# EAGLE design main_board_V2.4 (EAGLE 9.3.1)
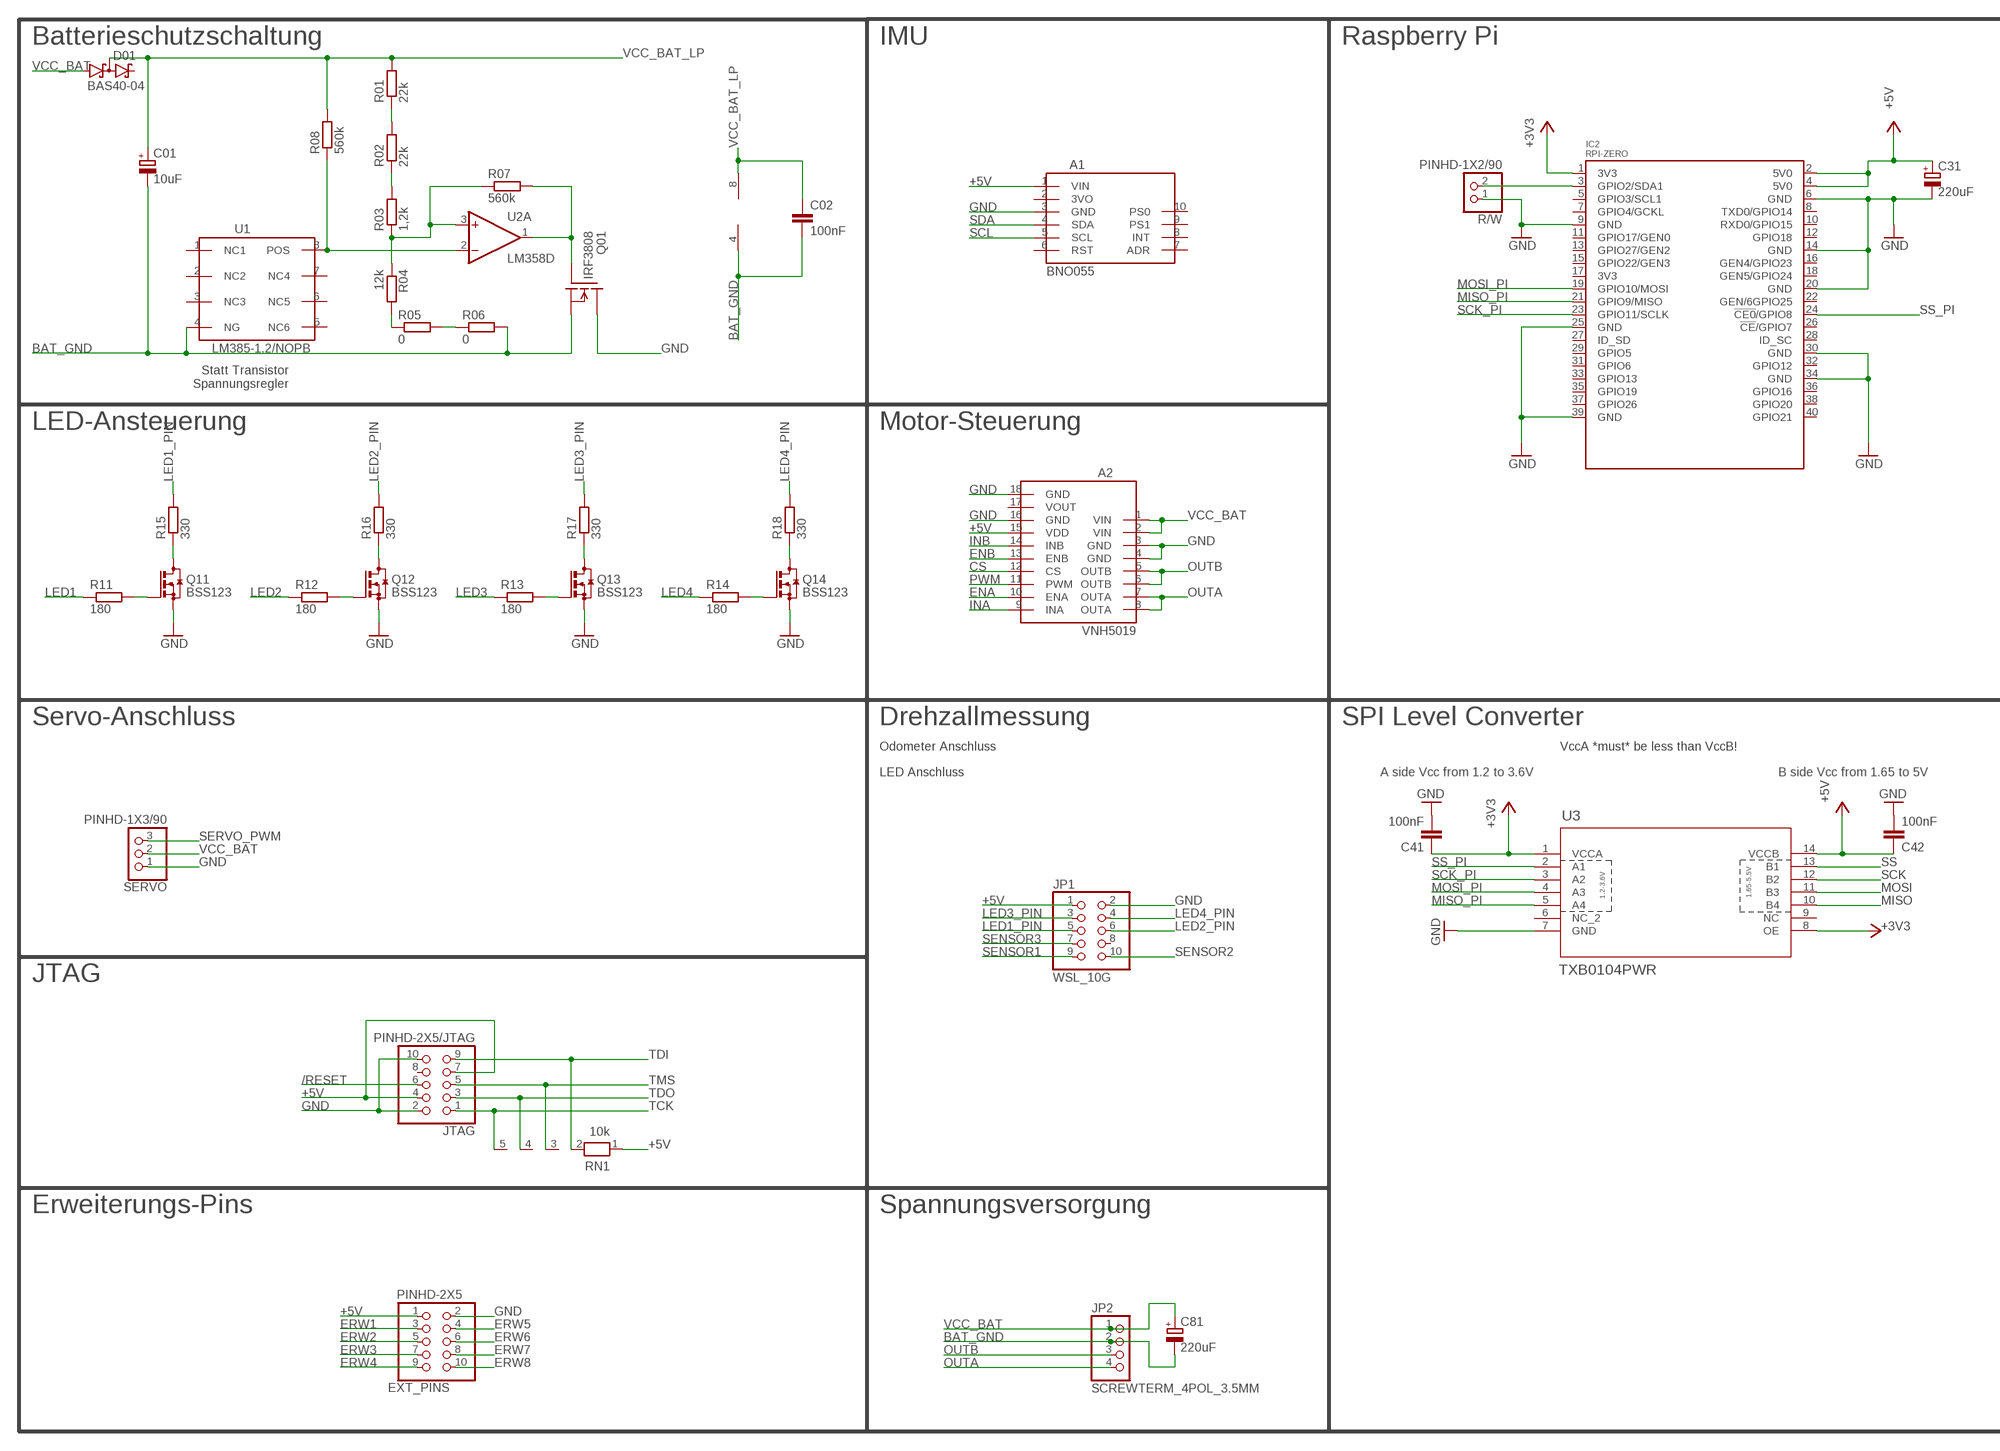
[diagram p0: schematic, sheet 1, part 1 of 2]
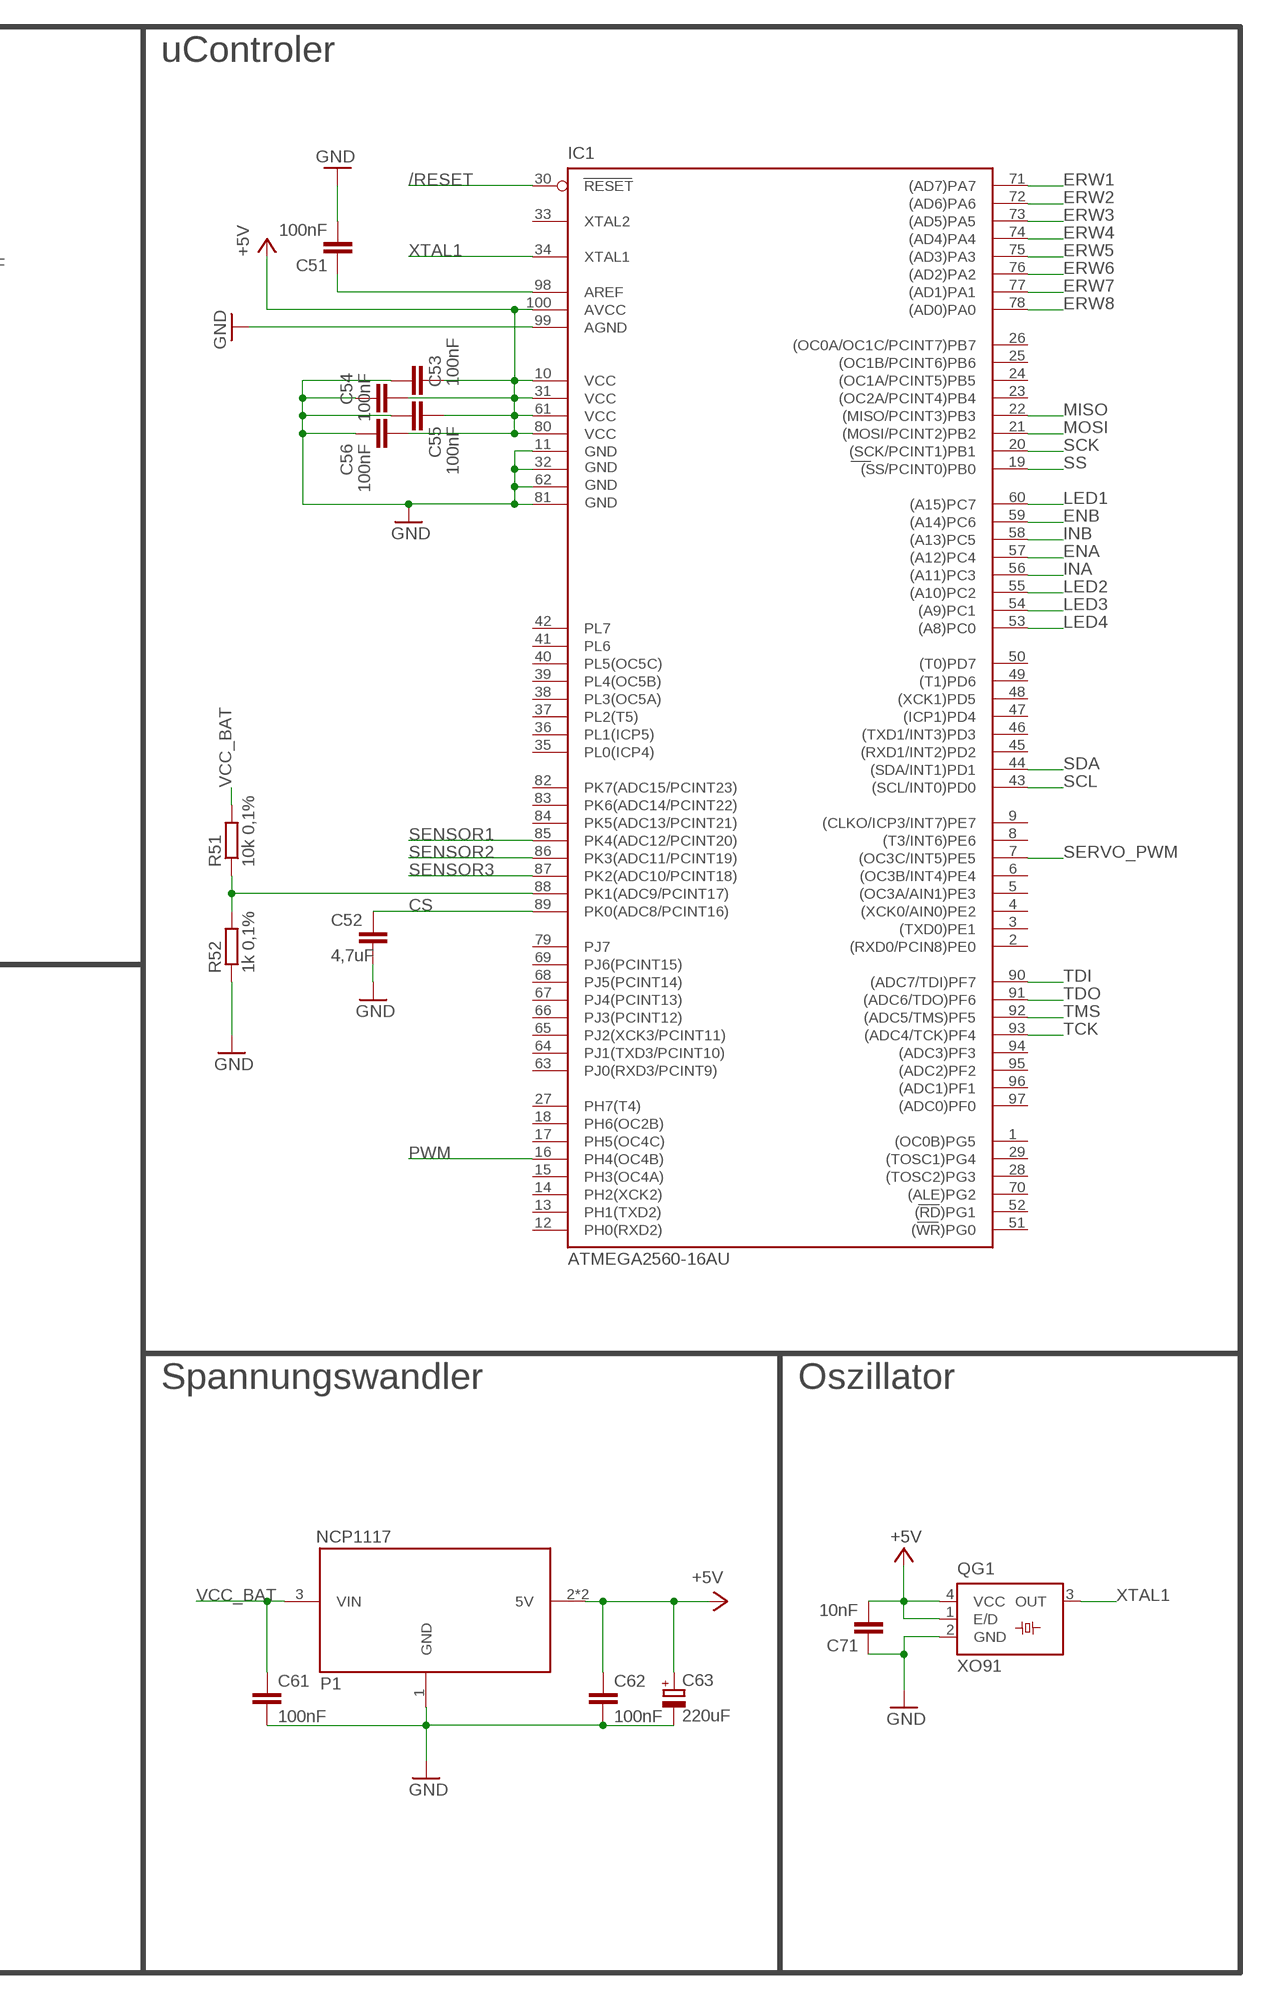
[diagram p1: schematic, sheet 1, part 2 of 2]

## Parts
A1  BNO055  [BNO055]
A2  VNH5019  [VNH5019]
C01  10uF  CPOL/4X5,8  [UD-4X5,8_NICHICON]
C02  100nF  C-EUC0805  [C0805]
C31  220uF  CPOL/6,3X7,7  [UD-6,3X5,8_NICHICON]
C41  100nF  C-EUC0805  [C0805]
C42  100nF  C-EUC0805  [C0805]
C51  100nF  C-EUC0805  [C0805]
C52  4,7uF  C-EUC0805  [C0805]
C53  100nF  C-EUC0805  [C0805]
C54  100nF  C-EUC0805  [C0805]
C55  100nF  C-EUC0805  [C0805]
C56  100nF  C-EUC0805  [C0805]
C61  100nF  C-EUC0805  [C0805]
C62  100nF  C-EUC0805  [C0805]
C63  220uF  CPOL/6,3X7,7  [UD-6,3X5,8_NICHICON]
C71  10nF  C-EUC0805  [C0805]
C81  220uF  CPOL/6,3X7,7  [UD-6,3X5,8_NICHICON]
D01  BAS40-04  [SOT23]
EXT_PINS  PINHD-2X5  [2X05]
IC1  ATMEGA2560-16AU  [TQFP100]
IC2  RPI-ZERO  [RASPBERRYPI_ZERO]
JP1  WSL_10G  [WSL_10G]
JP2  SCREWTERM_4POL_3.5MM  [SCREWTERM_4POS_3.5MM]
JTAG  PINHD-2X5/JTAG  [2X05/JTAG]
P1  NCP1117  [SOT223]
Q01  IRF3808  [TO220]
Q11  BSS123  [SOT23]
Q12  BSS123  [SOT23]
Q13  BSS123  [SOT23]
Q14  BSS123  [SOT23]
QG1  XO91  [SM77H]
R01  22k  R-EUR0805  [R0805]
R02  22k  R-EUR0805  [R0805]
R03  1,2k  R-EUR0805  [R0805]
R04  12k  R-EUR0805  [R0805]
R05  0  R-EUR0805  [R0805]
R06  0  R-EUR0805  [R0805]
R07  560k  R-EUR0805  [R0805]
R08  560k  R-EUR0805  [R0805]
R11  180  R-EUR0805  [R0805]
R12  180  R-EUR0805  [R0805]
R13  180  R-EUR0805  [R0805]
R14  180  R-EUR0805  [R0805]
R15  330  R-EUR0805  [R0805]
R16  330  R-EUR0805  [R0805]
R17  330  R-EUR0805  [R0805]
R18  330  R-EUR0805  [R0805]
R51  10k 0,1%  R-EUR0805  [R0805]
R52  1k 0,1%  R-EUR0805  [R0805]
R/W  PINHD-1X2/90  [1X02/90]
RN1  10k  RN04  [RN04]
SERVO  PINHD-1X3/90  [1X03/90]
U1  LM385-1.2/NOPB  [SO08]
U2  LM358D  [SO08]
U3  TXB0104PWR  [PW14]

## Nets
+3V3: C41.1 IC2.1(3V3) U3.1(VCCA) U3.8(OE)
+5V: A1.1(VIN) A2.15(VDD) C31.+ C42.1 C53.1 C54.1 C55.1 C56.1 C62.1 C63.+ C71.2 EXT_PINS.1 IC1.10(VCC) IC1.31(VCC1) IC1.61(VCC2) IC1.80(VCC3) IC1.100(AVCC) IC2.2(5V0) IC2.4(5V0) JP1.1 JTAG.4 JTAG.7 P1.2(5V) P1.4(5V) QG1.1(E/D) QG1.4(VCC) RN1.1 U3.14(VCCB)
/RESET: IC1.30(RESET) JTAG.6
BAT_GND: C01.- C02.2 C81.- JP2.2 Q01.3(S) R06.2 U1.4(NG) U2.4(P:V-)
CS: A2.12(CS) C52.1 IC1.89(PK0(ADC8/PCINT16))
ENA: A2.10(ENA) IC1.57((A12)PC4)
ENB: A2.13(ENB) IC1.59((A14)PC6)
ERW1: EXT_PINS.3 IC1.71((AD7)PA7)
ERW2: EXT_PINS.5 IC1.72((AD6)PA6)
ERW3: EXT_PINS.7 IC1.73((AD5)PA5)
ERW4: EXT_PINS.9 IC1.74((AD4)PA4)
ERW5: EXT_PINS.4 IC1.75((AD3)PA3)
ERW6: EXT_PINS.6 IC1.76((AD2)PA2)
ERW7: EXT_PINS.8 IC1.77((AD1)PA1)
ERW8: EXT_PINS.10 IC1.78((AD0)PA0)
GND: A1.3(GND) A2.3(GND) A2.4(GND) A2.16(GND) A2.18(GND) C31.- C41.2 C42.2 C51.2 C52.2 C53.2 C54.2 C55.2 C56.2 C61.2 C62.2 C63.- C71.1 EXT_PINS.2 IC1.11(GND) IC1.32(GND1) IC1.62(GND2) IC1.81(GND3) IC1.99(AGND) IC2.6(GND) IC2.9(GND) IC2.14(GND) IC2.20(GND) IC2.25(GND) IC2.30(GND) IC2.34(GND) IC2.39(GND) JP1.2 JTAG.2 JTAG.10 P1.1(GND) Q01.2(D) Q11.2(S) Q12.2(S) Q13.2(S) Q14.2(S) QG1.2(GND) R52.1 R/W.1 SERVO.1 U3.7(GND)
INA: A2.9(INA) IC1.56((A11)PC3)
INB: A2.14(INB) IC1.58((A13)PC5)
LED1: IC1.60((A15)PC7) R11.1
LED1_PIN: JP1.5 R15.2
LED2: IC1.55((A10)PC2) R12.1
LED2_PIN: JP1.6 R16.2
LED3: IC1.54((A9)PC1) R13.1
LED3_PIN: JP1.3 R17.2
LED4: IC1.53((A8)PC0) R14.1
LED4_PIN: JP1.4 R18.2
MISO: IC1.22((MISO/PCINT3)PB3) U3.10(B4)
MISO_PI: IC2.21(GPIO9/MISO) U3.5(A4)
MOSI: IC1.21((MOSI/PCINT2)PB2) U3.11(B3)
MOSI_PI: IC2.19(GPIO10/MOSI) U3.4(A3)
N$1: R05.2 R06.1
N$2: R03.1 R04.1 R07.1 U2.3(A:+IN)
N$3: R08.1 U1.8(POS) U2.2(A:-IN)
N$5: R01.1 R02.2
N$6: Q01.1(G) R07.2 U2.1(A:OUT)
N$7: R02.1 R03.2
N$8: IC2.3(GPIO2/SDA1) R/W.2
N$9: Q11.1(G) R11.2
N$10: Q12.1(G) R12.2
N$11: C51.1 IC1.98(AREF)
N$12: R04.2 R05.1
N$13: Q13.1(G) R13.2
N$14: Q14.1(G) R14.2
N$18: Q11.3(D) R15.1
N$19: Q12.3(D) R16.1
N$26: Q13.3(D) R17.1
N$29: Q14.3(D) R18.1
N$30: IC1.88(PK1(ADC9/PCINT17)) R51.1 R52.2
OUTA: A2.7(OUTA) A2.8(OUTA) JP2.4
OUTB: A2.5(OUTB) A2.6(OUTB) JP2.3
PWM: A2.11(PWM) IC1.16(PH4(OC4B))
SCK: IC1.20((SCK/PCINT1)PB1) U3.12(B2)
SCK_PI: IC2.23(GPIO11/SCLK) U3.3(A2)
SCL: A1.5(SCL) IC1.43((SCL/INT0)PD0)
SDA: A1.4(SDA) IC1.44((SDA/INT1)PD1)
SENSOR1: IC1.85(PK4(ADC12/PCINT20)) JP1.9
SENSOR2: IC1.86(PK3(ADC11/PCINT19)) JP1.10
SENSOR3: IC1.87(PK2(ADC10/PCINT18)) JP1.7
SERVO_PWM: IC1.7((OC3C/INT5)PE5) SERVO.3
SS: IC1.19((SS/PCINT0)PB0) U3.13(B1)
SS_PI: IC2.24(!CE0!/GPIO8) U3.2(A1)
TCK: IC1.93((ADC4/TCK)PF4) JTAG.1 RN1.5
TDI: IC1.90((ADC7/TDI)PF7) JTAG.9 RN1.2
TDO: IC1.91((ADC6/TDO)PF6) JTAG.3 RN1.4
TMS: IC1.92((ADC5/TMS)PF5) JTAG.5 RN1.3
VCC_BAT: A2.1(VIN) A2.2(VIN) C61.1 C81.+ D01.1(A1) JP2.1 P1.3(VIN) R51.2 SERVO.2
VCC_BAT_LP: C01.+ C02.1 D01.3(C1A2) R01.2 R08.2 U2.8(P:V+)
XTAL1: IC1.34(XTAL1) QG1.3(OUT)
Unconnected: A1.2(3VO) A1.6(RST) A1.7(ADR) A1.8(INT) A1.9(PS1) A1.10(PS0) A2.17(VOUT) D01.2(C2) IC1.1((OC0B)PG5) IC1.2((RXD0/PCIN8)PE0) IC1.3((TXD0)PE1) IC1.4((XCK0/AIN0)PE2) IC1.5((OC3A/AIN1)PE3) IC1.6((OC3B/INT4)PE4) IC1.8((T3/INT6)PE6) IC1.9((CLKO/ICP3/INT7)PE7) IC1.12(PH0(RXD2)) IC1.13(PH1(TXD2)) IC1.14(PH2(XCK2)) IC1.15(PH3(OC4A)) IC1.17(PH5(OC4C)) IC1.18(PH6(OC2B)) IC1.23((OC2A/PCINT4)PB4) IC1.24((OC1A/PCINT5)PB5) IC1.25((OC1B/PCINT6)PB6) IC1.26((OC0A/OC1C/PCINT7)PB7) IC1.27(PH7(T4)) IC1.28((TOSC2)PG3) IC1.29((TOSC1)PG4) IC1.33(XTAL2) IC1.35(PL0(ICP4)) IC1.36(PL1(ICP5)) IC1.37(PL2(T5)) IC1.38(PL3(OC5A)) IC1.39(PL4(OC5B)) IC1.40(PL5(OC5C)) IC1.41(PL6) IC1.42(PL7) IC1.45((RXD1/INT2)PD2) IC1.46((TXD1/INT3)PD3) IC1.47((ICP1)PD4) IC1.48((XCK1)PD5) IC1.49((T1)PD6) IC1.50((T0)PD7) IC1.51((WR)PG0) IC1.52((RD)PG1) IC1.63(PJ0(RXD3/PCINT9)) IC1.64(PJ1(TXD3/PCINT10)) IC1.65(PJ2(XCK3/PCINT11)) IC1.66(PJ3(PCINT12)) IC1.67(PJ4(PCINT13)) IC1.68(PJ5(PCINT14)) IC1.69(PJ6(PCINT15)) IC1.70((ALE)PG2) IC1.79(PJ7) IC1.82(PK7(ADC15/PCINT23)) IC1.83(PK6(ADC14/PCINT22)) IC1.84(PK5(ADC13/PCINT21)) IC1.94((ADC3)PF3) IC1.95((ADC2)PF2) IC1.96((ADC1)PF1) IC1.97((ADC0)PF0) IC2.5(GPIO3/SCL1) IC2.7(GPIO4/GCKL) IC2.8(TXD0/GPIO14) IC2.10(RXD0/GPIO15) IC2.11(GPIO17/GEN0) IC2.12(GPIO18) IC2.13(GPIO27/GEN2) IC2.15(GPIO22/GEN3) IC2.16(GEN4/GPIO23) IC2.17(3V3) IC2.18(GEN5/GPIO24) IC2.22(GEN/6GPIO25) IC2.26(!CE!/GPIO7) IC2.27(ID_SD) IC2.28(ID_SC) IC2.29(GPIO5) IC2.31(GPIO6) IC2.32(GPIO12) IC2.33(GPIO13) IC2.35(GPIO19) IC2.36(GPIO16) IC2.37(GPIO26) IC2.38(GPIO20) IC2.40(GPIO21) JP1.8 JTAG.8 U1.1(NC1) U1.2(NC2) U1.3(NC3) U1.5(NC6) U1.6(NC5) U1.7(NC4) U2.5(B:+IN) U2.6(B:-IN) U2.7(B:OUT) U3.6(NC_2) U3.9(NC)

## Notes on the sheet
- Batterieschutzschaltung | IMU | Raspberry Pi | uControler
- Statt Transistor
  Spannungsregler
- LED-Ansteuerung | Motor-Steuerung
- Servo-Anschluss | Drehzallmessung | SPI Level Converter
- Odometer Anschluss | VccA *must* be less than VccB!
- LED Anschluss | A side Vcc from 1.2 to 3.6V | B side Vcc from 1.65 to 5V
- JTAG
- Spannungswandler | Oszillator
- Erweiterungs-Pins | Spannungsversorgung

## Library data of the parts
A1 = embedded:BNO055: BREAKOUT BOARD Adafruit BNO055 Absolute Orientation Sensor https://learn.adafruit.com/adafruit-bno055-absolute-orientation-sensor/overview; DATASHEET: https://cdn-learn.adafruit.com/downloads/pdf/adafruit-bno055-absolute-orientation-sensor.pdf; DESCR: Acceleration Sensor Development Tools Adafruit 9-DOF Absolute Orientation IMU Fusion Breakout - BNO055; MF: Adafruit; MF_PN: 2472; MOUSER_NO: 485-2472; PURCHASE: https://www.reichelt.de/development-boards-sensor-with-different-functions-debo-sens-combi-p235479.html?PROVID=2788&gclid=EAIaIQobChMIppaP2Nqd4gIVA853Ch3mIQILEAYYASABEgKn7_D_BwE&&r=1; REICHELT_NO: DEBO SENS COMBI; UNIT_PRICE: 30.52
A2 = embedded:VNH5019: Pololu VNH5019 Motor Driver Carrier Operating voltage: 5.5 – 24 V1 Output current: 12 A continuous (30 maximum) 3V-compatible inputs PWM operation up to 20 kHz, which is ultrasonic and allows for quieter motor operation Current sense output proportional to motor current (approx. 140 mV/A; only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; DATASHEET: https://www.st.com/content/ccc/resource/technical/document/data_brief/3b/bf/c3/13/d5/b2/4c/b0/DM00101248.pdf/files/DM00101248.pdf/jcr:content/translations/en.DM00101248.pdf; DESCR: VNH5019 Motor Controller/Driver Power Management Evaluation Board; DIGIKEY_NO: 497-14839-ND; MF: Pololu; MF_PN: 1451; PURCHASE: https://www.digikey.de/product-detail/de/stmicro/EVAL-VNH5019-P1/497-14839-ND/4869482?utm_adgroup=Dev+Boards+and+Kits&mkwid=siS2m191I&pcrid=218211101233&pkw=&pmt=&pdv=c&productid=4869482&slid=&gclid=CjwKCAjw2cTmBRAVEiwA8YMgzaipRkISnCfVdTSSKNDcojFwUwpzQeKwWGZWYQUEEXtJxoFNqy7q1BoC5-sQAvD_BwE; UNIT_PRICE: 33.42
C01 = embedded:CPOL: Aluminum Electrolytic Capacitors; DATASHEET: https://industrial.panasonic.com/cdbs/www-data/pdf/RDE0000/ABA0000C1175.pdf; DESCR: Aluminium Electrolytic Capacitors - SMD FK 35VDC 10uF SMD 4x5.8; FARNELL_NO: 1244420; MF: Panasonic; MF_PN: EEEFKV100UAR; PACKAGE: 4x5.8; PURCHASE: https://de.farnell.com/panasonic/eeefkv100uar/kondensator-10-f-35v-radial-smd/dp/1244420; SIZE: 4x5.8mm; UNIT_PRICE: 0.376
C02 C41 C42 C51-C56 C61 C62 C71 = embedded:C-EU: Capacitor; DESCR: SMD Capacitor; PACKAGE: C0805; SIZE: 0805in
C31 C63 C81 = embedded:CPOL: Aluminum Electrolytic Capacitors; DATASHEET: https://industrial.panasonic.com/cdbs/www-data/pdf/RDE0000/ABA0000C1175.pdf; DESCR: Aluminium Electrolytic Capacitors - SMD FK 16VDC 10uF SMD 6.3x7.7; FARNELL_NO: 2254321; MF: Panasonic; MF_PN: EEEFKC221XAP; PACKAGE: 6.3x7.7; PURCHASE: https://de.farnell.com/panasonic/eeefkc221xap/kondensator-220-f-16v-radial-smd/dp/2254321; SIZE: 6.3x7.7mm; UNIT_PRICE: 0.48
D01 = embedded:BAS40-04: Silicon Schottky Diodes General-purpose diode for high-speed switching; DATASHEET: https://www.onsemi.com/pub/Collateral/BAS40-04LT1-D.PDF; DESCR: Schottky Diodes & Rectifiers 40V 225mW Dual; FARNELL_NO: 2317418; MF: ON Semiconductor; MF_PN: BAS40-04LT1G; MOUSER_NO: 863-BAS40-04LT1G; PACKAGE: SOT-23-3; PURCHASE: https://de.farnell.com/on-semiconductor/bas40-04lt1g/schottky-diode-40ma-40v-sot-23/dp/2317418; UNIT_PRICE: 0.236
EXT_PINS = embedded:PINHD-2X5: PIN HEADER; ANGLE: Straight; DESCR: Pin Header 2X5 0DEG; PACKAGE: Pin Header; PITCH: 2.54mm; POS: 10; ROWS: 2
IC1 = embedded:ATMEGA*: MICROCONTROLLER 64/128/256 Kbytes FLASH 4 Kbytes EEPROM 8 Kbytes SRAM 86 General Purpose I/O pins 12-channels16-bit PWM 4 x Serial USARTs 16-channels 10-bit A/D; DATASHEET: http://ww1.microchip.com/downloads/en/DeviceDoc/Atmel-2549-8-bit-AVR-Microcontroller-ATmega640-1280-1281-2560-2561_datasheet.pdf; DESCR: 8-bit Microcontrollers - MCU 256kB Flash 4kB EEPROM 86 I/O Pins; FARNELL_NO: 1288330; MF: Atmel; MF_PN: ATMEGA2560-16AU; MOUSER_NO: 556-ATMEGA2560-16AU; PACKAGE: TQFP-100; PURCHASE: https://de.farnell.com/atmel/atmega2560-16au/8bit-mcu-256k-flash-5v-smd-2560/dp/1288330; UNIT_PRICE: 10.13
IC2 = embedded:RPI-ZERO: Raspberry Pi Zero W BCM 2835 SOC @ 1GHz 1GHz 512MB of RAM On-board Wireless LAN - 2.4 GHz 802.11 b/g/n (BCM43438) On-board Bluetooth 4.1 + HS Low-energy (BLE) (BCM43438) micro-SD mini-HDMI micro-B USB for data micro-B USB for power CSI camera connector (needs adaptor cable) Unpopulated 40-pin GPIO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; DESCR: Raspberry Pi Zero W; MF: Raspberry Pi; UNIT_PRICE: 10.53
JP1 = embedded:WSL_10G: Connector WSL 10G WANNENSTECKER, 10-POLIG BOX HEADER Source: Box Header; ANGLE: Straight; DATASHEET: https://cdn-reichelt.de/documents/datenblatt/C151/BH1S-XX-L.pdf; DESCR: Box connector 10pin straight; MF: Amtek; MF_PN: WSL-10G; PACKAGE: Box Header; PITCH: 2.54mm; POS: 10; PURCHASE: https://www.reichelt.de/box-connector-10-pin-straight-wsl-10g-p22816.html?r=1; REICHELT_NO: WSL 10G; ROWS: 2; UNIT_PRICE: 0.1
JP2 = embedded:SCREWTERM_4POL_3.5MM: Plug-In Screw Terminal Connector 2 Part Plug-InScrew Terminal 4 position 3.5mm pitch table, th, td { padding: 5px; } th { text-align: left; } table { } Plug Pin Header AKL 166-04 STL 224-04 Datasheet Datasheet; ANGLE: 90; DATASHEET: https://cdn-reichelt.de/documents/datenblatt/C100/31166102.pdf; https://cdn-reichelt.de/documents/datenblatt/C100/31224102.pdf; DESCR: Plug-in Connection Screw Terminal 4P 3.5mm 90DEG; Pin Header for Terminal 4P 3.5 mm; MF: RIACON; MF_PN: AKL 166-04; STL 224-04; PACKAGE: Screw Terminal; Pin Header for Terminal; PITCH: 3.50mm; POS: 4; PURCHASE: https://www.reichelt.com/de/en/plug-in-connection-terminal-4-pin-spacing-3-5-mm-akl-166-04-p72073.html?&trstct=pos_9; https://www.reichelt.com/de/en/pin-header-for-terminal-4-pin-spacing-3-5-mm-stl-224-04-p72080.html?&trstct=pos_0; REICHELT_NO: AKL 166-04; STL 224-04; ROWS: 1; UNIT_PRICE: 0.95; 0.34
JTAG = embedded:PINHD-2X5: PIN HEADER; ANGLE: Straight; DESCR: Pin Header 2X5 0DEG JTAG; PACKAGE: Pin Header; PITCH: 2.54mm; POS: 10; ROWS: 2
P1 = embedded:NCP1117: Voltage Regulator NCP1117 1.0A 5.0V Low-Dropout Positive Fixed and Adjustable Voltage Regulators ON Semiconductor; DATASHEET: https://www.mouser.de/datasheet/2/308/NCP1117-D-81326.pdf; DESCR: LDO Voltage Regulators 5.0V 1A Positive - SOT-223-3; FARNELL_NO: 2112617; MF: ON Semiconductor; MF_PN: NCP1117ST50T3G; MOUSER_NO: 863-NCP1117ST50T3G; PACKAGE: SOT-223-3; PURCHASE: https://de.farnell.com/on-semiconductor/ncp1117st50t3g/ldo-reg-15vin-1a-5v-1-3sot223/dp/2112617; UNIT_PRICE: 0.41
Q01 = embedded:IRF3808: MOSFET N-Channel Enhancement MOSFET (HEXFET); 75V; 140A; 0,007Ohm; DATASHEET: https://www.mouser.de/datasheet/2/427/sihf510-105610.pdf; DESCR: MOSFET N-CH 75V HEXFET MOSFET D2-PA; FARNELL_NO: 1653658; MF: Vishay; MF_PN: IRF3808PBF; MOUSER_NO: 942-IRF3808PBF; PACKAGE: TO-220AB; PURCHASE: https://de.farnell.com/infineon/irf3808pbf/mosfet-n-kanal-75v-140a-to-220/dp/8657661; UNIT_PRICE: 1.55
Q11-Q14 = embedded:BSS123: MOSFET N-Channel MOSFET; DATASHEET: https://www.onsemi.com/pub/Collateral/BSS123-D.PDF; DESCR: MOSFET SOT-23 N-CH LOGIC; FARNELL_NO: 9845330; MF: ON Semiconductor; MF_PN: BSS123; MOUSER_NO: 512-BSS123; PACKAGE: SOT-23-3; PURCHASE: https://de.farnell.com/on-semiconductor/bss123/mosfet-n-kanal-100v-sot-23/dp/9845321; UNIT_PRICE: 0.236
QG1 = embedded:XO91: Oscillator 3.3V CMOS Clock Oscillator Source: Datasheet; DATASHEET: https://cdn-reichelt.de/documents/datenblatt/B400/XO91.pdf; DESCR: 16.0MHz CMOS Crystal Oscillator Ceramic SMD XO91; FREQUENCY: 16MHz; MF: EUROQUARTZ; MF_PN: 16.000MHZ XO91050UITA; PACKAGE: 7x5; PURCHASE: https://www.reichelt.de/16-0mhz-crystal-oscillator-ceramic-smd-xo91-xo91-16-00000-p85017.html?&trstct=pol_12; REICHELT_NO: XO91 16,00000; SIZE: 7x5mm; UNIT_PRICE: 1.15
R01-R08 R11-R18 R51 R52 = embedded:R-EU: Resistor; DESCR: SMD Resistor; PACKAGE: C0805; SIZE: 0805in
R/W = embedded:PINHD-1X2: PIN HEADER; ANGLE: 90; DESCR: Pin Header 1X2 90DEG; PACKAGE: Pin Header; PITCH: 2.54mm; POS: 2; ROWS: 1
RN1 = embedded:RN04: RESISTOR NETWORK A resistor network is a single package that contains two or more resistors. The package will include multiple leads by which the network can be made part of a larger circuit. Figure 7 shows typical packages used for resistor networks. There are commonly two ways the resistors are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; DATASHEET: https://www.bourns.com/pdfs/4600X.pdf; DESCR: Resistor Networks & Arrays 5pin 4resistor 10Kohms 2% Bussed; FARNELL_NO: 9356061; MF: Bourns; MF_PN: 4605X-101-103LF; PACKAGE: SIP; POS: 5; PURCHASE: https://de.farnell.com/bourns/4605x-101-103lf/widerstandsnetzwerk-5-pins-10k/dp/9356061; RES: 4; UNIT_PRICE: 0.294
SERVO = embedded:PINHD-1X3: PIN HEADER; ANGLE: 90; PACKAGE: Pin Header; PITCH: 2.54mm; POS: 3; ROWS: 1
U1 = embedded:LM385-1.2/NOPB: Voltage Ref LM385M Texas Instruments; DATASHEET: http://www.ti.com/lit/ds/symlink/lm385-1.2-n.pdf; DESCR: Voltage References Fixed 1.235 MicroPwr Vtg Ref - SOIC-8; FARNELL_NO: 2782470; MF: Texas Instruments; MF_PN: LM385MX-1.2/NOPB; PACKAGE: SOIC-8; PURCHASE: https://de.farnell.com/texas-instruments/lm385mx-1-2-nopb/spannungsreferenz-shunt-1-235v/dp/2782470; UNIT_PRICE: 0.60
U2 = embedded:LM358: OP AMP also LM158; LM258; LM2904 Source: Datasheet; DATASHEET: http://www.ti.com/lit/ds/symlink/lm358.pdf; DESCR: Operational Amplifiers - Op Amps Dual Linear - SOIC-8; FARNELL_NO: 1648685; MF: Texas Instruments; MF_PN: LM358D; MOUSER_NO: 595-LM358D; PACKAGE: SOIC-8; PURCHASE: https://de.farnell.com/texas-instruments/lm358dr/op-amp-dual-low-power-soic8-358/dp/1648685; UNIT_PRICE: 0.358
U3 = embedded:TXB0104PWR: Level Translator Voltage Levels 4-Bit Bi-directional V-Level Translator Hook-Up Guide: TXB0104 Level Shifter Hookup Guide; DATASHEET: http://www.ti.com/lit/ds/symlink/txb0104.pdf; DESCR: Translation - Voltage Levels 4-Bit Bi-directional V-Level Translator; FARNELL_NO: 1607891; MF: Texas Instruments; MF_PN: TXB0104PWR; MOUSER_NO: 595-TXB0104PWR; PACKAGE: TSSOP-14; PURCHASE: https://de.farnell.com/texas-instruments/txb0104pwr/ic-sm-logik-translator/dp/1607891; UNIT_PRICE: 1.11

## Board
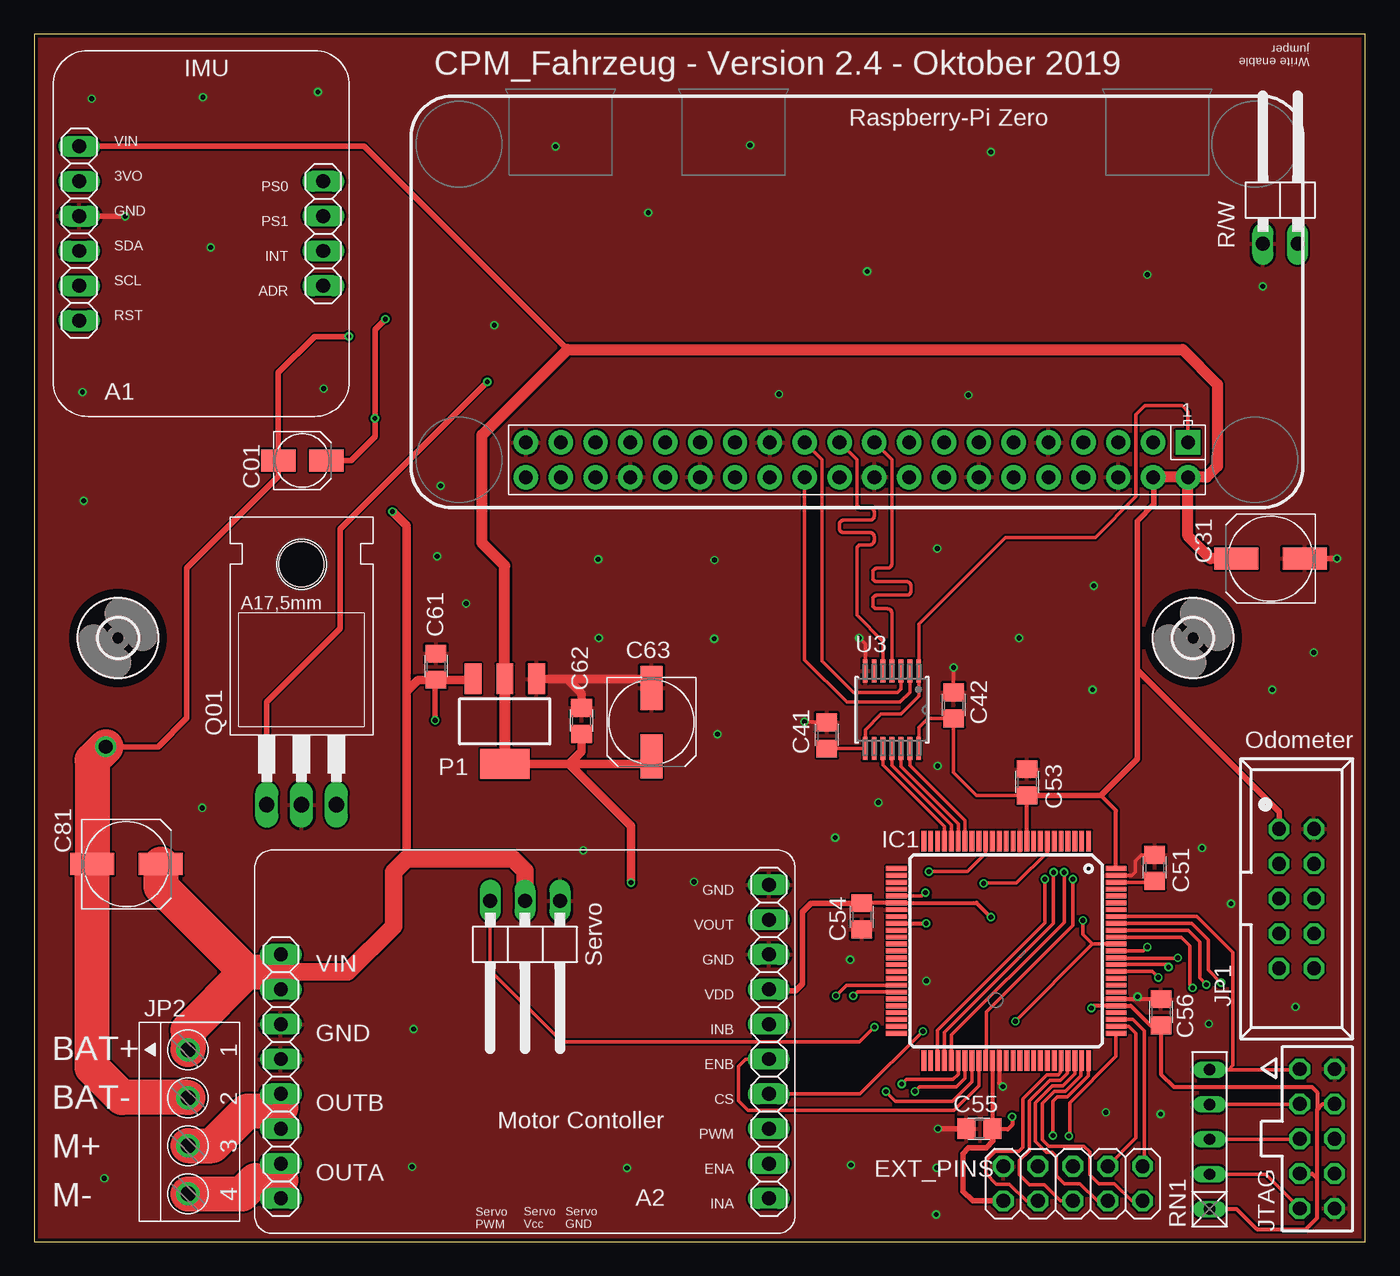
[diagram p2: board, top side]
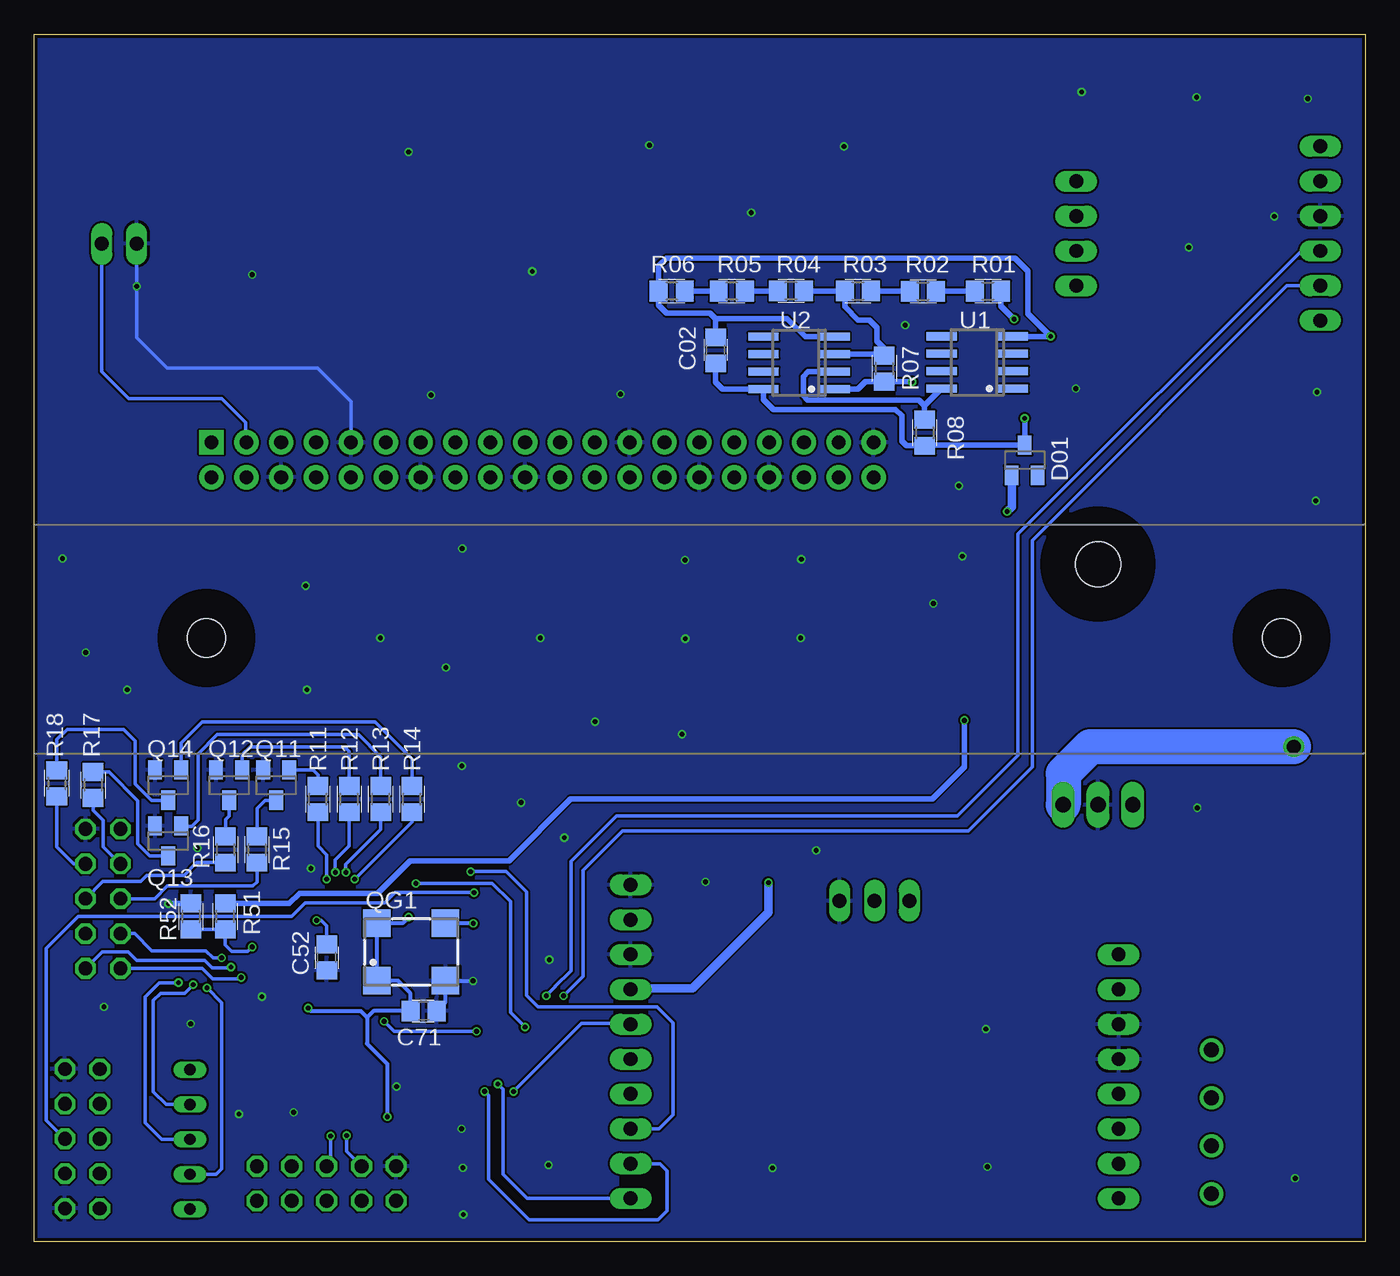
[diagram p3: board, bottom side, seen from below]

Size 97 x 88 mm. Coordinates in mm from the lower left corner, seen from the top.
Outline: 0,0 97,0 97,88 0,88 0,0
Copper layers (1*16): Top 0.018mm / dielectric 1.55mm / Bottom 0.018mm
Design rules "eC_2Layer_PClass6_BaseCopperO18_eCDefault *": minimum track width 0.15mm, minimum drill 0.35mm, track to track 0.15mm, track to pad 0.15mm, pad to pad 0.15mm, via to via 0.15mm, smd to smd 0mil, copper to edge 0.25mm, drill to drill 0.35mm, minimum pad ring 0.175mm, minimum via ring 0.125mm, stop-mask expansion 0mil, vias tented up to drill 0.45mm, thermal gap 0.2mm
bRestrict: area 54,4.2 to 54.3,4.8

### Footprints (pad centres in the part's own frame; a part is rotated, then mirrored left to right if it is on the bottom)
BNO055 = drill 1.016 long: 1 -8.89,6.35; 2 -8.89,3.81; 3 -8.89,1.27; 4 -8.89,-1.27; 5 -8.89,-3.81; 6 -8.89,-6.35; 7 8.89,-3.81; 8 8.89,-1.27; 9 8.89,1.27; 10 8.89,3.81
VNH5019 = drill 1.016 long: 1 -17.78,8.89; 2 -17.78,6.35; 3 -17.78,3.81; 4 -17.78,1.27; 5 -17.78,-1.27; 6 -17.78,-3.81; 7 -17.78,-6.35; 8 -17.78,-8.89; 9 17.78,-8.89; 10 17.78,-6.35; 11 17.78,-3.81; 12 17.78,-1.27; 13 17.78,1.27; 14 17.78,3.81; 15 17.78,6.35; 16 17.78,8.89; 17 17.78,11.43; 18 17.78,13.97
UD-4X5,8_NICHICON = smd 2.5 x 1.6: + 1.75,0; - -1.75,0
C0805 = smd 1.3 x 1.5: 1 -0.95,0; 2 0.95,0
UD-6,3X5,8_NICHICON = smd 3.2 x 1.6: + 2.5,0; - -2.5,0
SOT23 = smd 1 x 1.4: 1 -0.95,-1.1; 2 0.95,-1.1; 3 0,1.1
2X05 = drill 1.016 octagon: 1 -5.08,-1.27; 2 -5.08,1.27; 3 -2.54,-1.27; 4 -2.54,1.27; 5 0,-1.27; 6 0,1.27; 7 2.54,-1.27; 8 2.54,1.27; 9 5.08,-1.27; 10 5.08,1.27
TQFP100 = smd 1.5 x 0.35: 1 -8,6; 2 -8,5.5; 3 -8,5; 4 -8,4.5; 5 -8,4; 6 -8,3.5; 7 -8,3; 8 -8,2.5; 9 -8,2; 10 -8,1.5; 11 -8,1; 12 -8,0.5; 13 -8,0; 14 -8,-0.5; 15 -8,-1; 16 -8,-1.5; 17 -8,-2; 18 -8,-2.5; 19 -8,-3; 20 -8,-3.5; 21 -8,-4; 22 -8,-4.5; 23 -8,-5; 24 -8,-5.5; 25 -8,-6; 51 8,-6; 52 8,-5.5; 53 8,-5; 54 8,-4.5; 55 8,-4; 56 8,-3.5; 57 8,-3; 58 8,-2.5; 59 8,-2; 60 8,-1.5; 61 8,-1; 62 8,-0.5; 63 8,0; 64 8,0.5; 65 8,1; 66 8,1.5; 67 8,2; 68 8,2.5; 69 8,3; 70 8,3.5; 71 8,4; 72 8,4.5; 73 8,5; 74 8,5.5; 75 8,6 | smd 0.35 x 1.5: 26 -6,-8; 27 -5.5,-8; 28 -5,-8; 29 -4.5,-8; 30 -4,-8; 31 -3.5,-8; 32 -3,-8; 33 -2.5,-8; 34 -2,-8; 35 -1.5,-8; 36 -1,-8; 37 -0.5,-8; 38 0,-8; 39 0.5,-8; 40 1,-8; 41 1.5,-8; 42 2,-8; 43 2.5,-8; 44 3,-8; 45 3.5,-8; 46 4,-8; 47 4.5,-8; 48 5,-8; 49 5.5,-8; 50 6,-8; 76 6,8; 77 5.5,8; 78 5,8; 79 4.5,8; 80 4,8; 81 3.5,8; 82 3,8; 83 2.5,8; 84 2,8; 85 1.5,8; 86 1,8; 87 0.5,8; 88 0,8; 89 -0.5,8; 90 -1,8; 91 -1.5,8; 92 -2,8; 93 -2.5,8; 94 -3,8; 95 -3.5,8; 96 -4,8; 97 -4.5,8; 98 -5,8; 99 -5.5,8; 100 -6,8
RASPBERRYPI_ZERO = drill 1 pad 1.778 square: 1 8.37,25.23 | drill 1 pad 1.778: 2 8.37,27.77; 3 10.91,25.23; 4 10.91,27.77; 5 13.45,25.23; 6 13.45,27.77; 7 15.99,25.23; 8 15.99,27.77; 9 18.53,25.23; 10 18.53,27.77; 11 21.07,25.23; 12 21.07,27.77; 13 23.61,25.23; 14 23.61,27.77; 15 26.15,25.23; 16 26.15,27.77; 17 28.69,25.23; 18 28.69,27.77; 19 31.23,25.23; 20 31.23,27.77; 21 33.77,25.23; 22 33.77,27.77; 23 36.31,25.23; 24 36.31,27.77; 25 38.85,25.23; 26 38.85,27.77; 27 41.39,25.23; 28 41.39,27.77; 29 43.93,25.23; 30 43.93,27.77; 31 46.47,25.23; 32 46.47,27.77; 33 49.01,25.23; 34 49.01,27.77; 35 51.55,25.23; 36 51.55,27.77; 37 54.09,25.23; 38 54.09,27.77; 39 56.63,25.23; 40 56.63,27.77
WSL_10G = drill 1 octagon: 1 -5.08,-1.27; 2 -5.08,1.27; 3 -2.54,-1.27; 4 -2.54,1.27; 5 0,-1.27; 6 0,1.27; 7 2.54,-1.27; 8 2.54,1.27; 9 5.08,-1.27; 10 5.08,1.27
SCREWTERM_4POS_3.5MM = drill 1.1 pad 1.7: 1 -5.25,-0.1; 2 -1.75,-0.1; 3 1.75,-0.1; 4 5.25,-0.1
2X05/JTAG = drill 1 octagon: 1 -5.08,-1.27; 2 -5.08,1.27; 3 -2.54,-1.27; 4 -2.54,1.27; 5 0,-1.27; 6 0,1.27; 7 2.54,-1.27; 8 2.54,1.27; 9 5.08,-1.27; 10 5.08,1.27
SOT223 = smd 1.219 x 2.235: 1 -2.311,-3.099; 2 0,-3.099; 3 2.311,-3.099 | smd 3.6 x 2.2: 4 0,3.099
TO220 = drill 1.118 long: 1 -2.54,-6.35; 2 0,-6.35; 3 2.54,-6.35 | hole 3.302: 0,11.176
SM77H = smd 2 x 2: 1 -2.5,-2.1; 2 2.5,-2.1; 3 2.5,2.1; 4 -2.5,2.1
R0805 = smd 1.3 x 1.5: 1 -0.95,0; 2 0.95,0
1X02/90 = drill 1.016 long: 1 -1.27,-3.81; 2 1.27,-3.81
RN04 = drill 0.813 long: 1 -5.08,0; 2 -2.54,0; 3 0,0; 4 2.54,0; 5 5.08,0
1X03/90 = drill 1.016 long: 1 -2.54,-3.81; 2 0,-3.81; 3 2.54,-3.81
SO08 = smd 0.6 x 2.2: 1 -1.905,-2.6; 2 -0.635,-2.6; 3 0.635,-2.6; 4 1.905,-2.6; 5 1.905,2.6; 6 0.635,2.6; 7 -0.635,2.6; 8 -1.905,2.6
PW14 = smd 1.676 x 0.356: 1 -2.819,1.95; 2 -2.819,1.3; 3 -2.819,0.65; 4 -2.819,0; 5 -2.819,-0.65; 6 -2.819,-1.3; 7 -2.819,-1.95; 8 2.819,-1.95; 9 2.819,-1.3; 10 2.819,-0.65; 11 2.819,0; 12 2.819,0.65; 13 2.819,1.3; 14 2.819,1.95
2,8 = hole 2.8: 0,0

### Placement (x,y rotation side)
A1  12.17,73.48 0 top
A2  35.75,12.04 0 top
C01  19.53,56.93 0 top
C02  47.34,64.96 90 bottom
C31  90.11,49.78 180 top
C41  57.76,36.88 90 top
C42  67.01,39.09 90 top
C51  81.66,27.24 90 top
C52  75.68,20.72 270 bottom
C53  72.36,33.48 90 top
C54  60.31,23.72 270 top
C55  68.88,8.23 180 top
C56  82.12,16.73 90 top
C61  29.28,41.91 90 top
C62  39.89,37.96 90 top
C63  44.98,37.87 270 top
C71  68.62,16.81 180 bottom
C81  6.72,27.52 0 top
D01  24.82,56.96 0 bottom
EXT_PINS  75.7,4.24 0 top
IC1  70.84,21.2 270 top
IC2  92.46,83.49 180 top
JP1  92,25 270 top
JP2  11.3,8.74 270 top
JTAG  93.5,7.5 270 top
P1  34.29,37.92 180 top
Q01  19.48,38.2 0 top
Q11  79.38,33.27 180 bottom
Q12  82.8,33.27 180 bottom
Q13  87.25,29.21 180 bottom
Q14  87.25,33.27 180 bottom
QG1  69.53,21.11 0 bottom
R01  27.5,69.28 0 bottom
R02  32.23,69.27 0 bottom
R03  36.97,69.29 0 bottom
R04  41.85,69.3 180 bottom
R05  46.16,69.28 180 bottom
R06  50.55,69.28 180 bottom
R07  35.04,63.64 270 bottom
R08  32.11,58.96 270 bottom
R11  76.33,32.26 90 bottom
R12  74.04,32.26 90 bottom
R13  71.75,32.26 90 bottom
R14  69.47,32.26 90 bottom
R15  80.77,28.57 270 bottom
R16  83.06,28.57 270 bottom
R17  92.71,33.28 270 bottom
R18  95.37,33.41 270 bottom
R51  83.08,23.7 90 bottom
R52  85.59,23.7 270 bottom
R/W  90.81,76.55 0 top
RN1  85.65,7.46 90 top
SERVO  35.76,21.03 180 top
U1  28.27,64.08 90 bottom
U2  41.26,64.05 90 bottom
U3  62.51,38.76 270 top
U$3  [2,8]  6.1,44 0 top
U$4  [2,8]  84.45,44 0 top

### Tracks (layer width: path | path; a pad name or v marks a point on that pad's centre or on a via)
+3V3
  Top 0.254: IC2.1 84.09,60.52 83.67,60.94 80.92,60.94 80.29,60.3 80.29,54.3 77.32,51.33 70.79,51.33 64.46,45 U3.1 64.46,39.77 63.15,38.46 61.72,38.46 60.56,37.29 U3.8 60.55,35.93 C41.1
+5V  (via drill 0.35)
  Top 0.254: C53.1 68.66,32.53 67,34.19 C42.1 65.11,38.14 64.46,37.48 U3.14
  Top 0.305: IC1.10 72.34,32.51 C53.1 | v77.04,17.02 77.21,17.2 IC1.80 79.92,17.2 81.33,15.78 C56.1 82.12,12.21 83.06,11.28 93.12,11.28 93.5,10.9 93.5,9.63 | C55.1 | 93.5,4.6 93.5,1.73 92.69,0.91 89.1,0.91 87.64,2.38 RN1.1 | 93.5,4.6 93.5,9.63 | 93.5,4.6 93.14,4.96 JTAG.7 | 93.5,9.63 93.91,10.04 JTAG.4 | IC1.100 78.84,31.43 77.73,32.53 | v71.27,9.11 71.27,8.51 70.94,8.18 69.88,8.18 C55.1 | v69.72,23.65 68.67,24.7 IC1.31 60.33,24.7 C54.1 | IC1.61 C55.1
  Top 0.406: C54.1 56.62,24.67 55.97,24.02 55.97,18.79 55.47,18.29 53.63,18.29 A2.15 | 80.38,41.69 80.38,52.53 81.59,53.74 81.59,55.68 IC2.4 | C53.1 77.73,32.53 80.38,35.18 80.38,41.69 | 69.88,8.18 69.88,7.34 69.38,6.84 68.1,6.84 67.68,6.42 67.68,3.68 68.39,2.96 EXT_PINS.1 | 38.86,65.02 24.04,79.85 3.29,79.85 A1.1 | 80.38,41.69 90.73,31.33 JP1.1
  Top 0.61: 38.96,34.82 P1.4 | v43.5,26.16 43.5,30.29 38.96,34.82 | 38.96,34.82 38.99,34.82 | 38.99,34.82 44.44,34.82 C63.+ | C62.1 39.89,35.72 38.99,34.82
  Top 0.813: C31.+ 85.72,49.78 84.09,51.42 IC2.2 | IC2.2 85.44,55.72 86.23,56.52 86.23,62.48 83.69,65.02 38.86,65.02 32.63,58.79 32.63,50.93 34.29,49.28 P1.2 P1.4 | IC2.2 81.63,55.72 81.59,55.68
  Bottom 0.305: 72.74,16.35 72.74,14.43 71.27,12.96 v71.27,9.11 | 72.74,16.35 72.28,16.81 C71.2 69.58,18.09 70.5,19.01 QG1.1 QG1.4 70.16,23.21 v69.72,23.65 | 72.74,16.35 73.22,16.82 76.83,16.82 v77.04,17.02
  Bottom 0.61: v43.5,26.16 43.5,24 49.04,18.46 53.46,18.46 A2.15
/RESET  (via drill 0.35)
  Top 0.254: IC1.30 64.71,25.2 v64.96,25.44
  Bottom 0.254: JTAG.6 96.13,8.86 96.13,21.37 93.81,23.7 78.25,23.7 77.25,24.69 71.45,24.69 70.69,25.44 v64.96,25.44
BAT_GND  (via drill 0.35, 1)
  Top 0.406: v5.21,36.07 9.02,36.07 11.11,38.16 11.11,49.1 17.78,55.77 C01.- 17.78,63.33 20.43,65.98 v22.92,65.98
  Top 2.54: JP2.2 11.18,10.51 6.38,10.51 4.22,12.67 C81.- 4.22,35.08 v5.21,36.07
  Bottom 0.406: C02.2 47.34,67.28 | U2.4 40.81,65.96 42.13,67.28 47.34,67.28 | 47.34,67.28 47.76,67.69 50.93,67.69 51.5,68.26 51.5,68.27 R06.2 51.5,71.12 50.93,71.69 25.53,71.69 24.57,70.74 24.57,67.63 v22.92,65.98 25.66,65.98 U1.4
  Bottom 2.54: Q01.3 22.02,34.12 20.07,36.07 v5.21,36.07
CS  (via drill 0.35)
  Top 0.254: v76.43,23.42 76.43,22.39 77.13,21.7 | 77.13,21.7 IC1.89 | v64.77,15.34 v64.76,15.34 60.19,10.77 A2.12 | v71.5,16.07 77.13,21.7
  Bottom 0.254: C52.1 75.68,23.02 76.08,23.42 v76.43,23.42 | v71.5,16.07 70.77,15.34 v64.77,15.34
ENA  (via drill 0.35)
  Top 0.254: v64.19,10.95 64.51,11.27 67.19,11.27 67.84,11.92 IC1.57
  Bottom 0.254: v64.19,10.95 63.91,10.67 63.91,4.54 60.95,1.59 51.55,1.59 50.88,2.26 50.88,5.16 51.41,5.69 A2.10
ENB
  Top 0.254: A2.13 51.84,13.31 51.31,12.78 51.31,10.26 52.01,9.56 67.03,9.56 68.84,11.37 IC1.59
ERW1
  Top 0.254: IC1.71 74.79,13.15 74.79,12.33 74.63,12.17 73.81,12.17 72.04,10.4 72.04,6.88 71.75,6.59 70.05,6.59 69.34,5.88 69.34,4.99 70.14,4.19 71.07,4.19 72.29,2.97 EXT_PINS.3
ERW2
  Top 0.254: IC1.72 75.29,13.15 75.29,12.26 74.8,11.76 74.02,11.76 72.52,10.26 72.52,6.63 71.81,5.92 71.81,4.88 72.52,4.16 73.6,4.16 74.8,2.96 EXT_PINS.5
ERW3
  Top 0.254: IC1.73 75.84,12.22 74.96,11.35 74.18,11.35 72.96,10.13 72.96,7.3 73.77,6.5 74.21,6.5 74.49,6.22 74.49,4.81 75.06,4.23 76.22,4.23 77.48,2.96 EXT_PINS.7
ERW4
  Top 0.254: IC1.74 76.29,13.15 76.29,12.11 75.13,10.95 74.35,10.95 73.47,10.07 73.47,7.44 73.94,6.96 76.49,6.96 76.92,6.54 76.92,4.89 77.6,4.21 78.73,4.21 79.98,2.96 EXT_PINS.9
ERW5  (via drill 0.35)
  Top 0.254: IC1.75 76.84,12.08 75.3,10.54 74.56,10.54 74.23,10.21 v74.23,7.74
  Bottom 0.254: v74.23,7.74 74.23,6.58 EXT_PINS.4
ERW6  (via drill 0.35)
  Top 0.254: IC1.76 78.84,13.5 75.47,10.13 75.47,7.77 v75.4,7.7
  Bottom 0.254: v75.4,7.7 75.4,5.8 EXT_PINS.6
ERW7
  Top 0.254: IC1.77 79.76,15.7 80.29,15.17 80.29,7.55 EXT_PINS.8
ERW8
  Top 0.254: IC1.78 80.08,16.2 80.91,15.36 80.91,5.64 EXT_PINS.10
GND  (via drill 0.35)
  Top 0.254: U3.7 60.56,43.55 v60.12,43.99 | IC1.99 79.98,26.7 80.24,26.95 80.24,27.74 80.7,28.19 C51.2 | C42.2 v67,41.86 | C41.2 57.69,37.9 v56.13,37.9
  Top 0.305: IC1.62 70.34,11.55 v70.59,11.3 | IC1.81 80.25,17.7 v80.42,17.86 80.6,17.68 C56.2
  Top 0.406: v6.63,74.73 6.6,74.75 A1.3 | C55.2 v65.86,8.23 | C31.- v94.94,49.78
  Top 0.61: P1.1 38.81,41.02 | 38.81,41.02 44.33,41.02 C63.- | C62.2 39.89,39.95 38.81,41.02
  Bottom 0.254: R/W.1 89.55,69.63 v89.53,69.62 89.53,65.89 87.3,63.65 76.35,63.65 73.93,61.23 IC2.9
  Bottom 0.305: C71.1 67.03,17.46 QG1.2 65.04,19.01 v65.02,19
  Bottom 0.406: R52.1 v87.21,24.65 v87.22,24.64
  other vias: 3.61,54 27.53,5.46 33.53,66.8 65.84,34.67 5.11,4.62 85.12,28.7 76.83,27.2 29.62,55.09 12.24,31.62 41.1,49.73 49.56,43.94 43.21,5.36 65.76,5.38 65.74,1.98 78.11,9.42 91.92,17.12 90.22,40.23 93.24,42.95 77.22,47.8 71.78,43.99 77.14,40.23 81.13,70.48 69.72,79.43 60.71,70.71 52.17,79.91 4.19,83.31 20.68,83.79 3.51,61.93 21.08,62.18 12.85,72.47 38,79.83 12.29,83.41 44.75,75.01 41.15,43.99 49.58,49.68 65.81,50.52 48.08,26.21 49.78,36.98 61.52,32 58.37,29.44 59.46,20.55 27.64,15.49 59.51,5.59 29.36,49.96 31.47,46.51 54.28,61.77 68.07,61.7 40.01,28.52 82.09,9.3 85.6,15.88
  pour Top: 0.18,87.85 96.85,87.85 96.85,0.13 0.16,0.13 0.16,87.84
  pour Bottom: 0.17,87.75 96.81,87.75 96.81,0.18 0.17,0.18 0.17,87.8
INA  (via drill 0.35)
  Top 0.254: IC1.56 67.34,12.21 66.96,11.84 63.58,11.84 v63.22,11.48
  Bottom 0.254: v63.22,11.48 62.84,11.1 62.84,4.92 61.07,3.15 A2.9
INB  (via drill 0.35)
  Top 0.254: v62.06,10.94 v62.06,10.93 62.77,10.23 66.92,10.23 68.34,11.64 IC1.58
  Bottom 0.254: v62.06,10.94 57.11,15.89 53.58,15.89 A2.14
LED1  (via drill 0.35)
  Top 0.254: v75.69,26.42 75.69,23.06 69.38,16.75 69.38,13.24 IC1.60
  Bottom 0.254: v75.69,26.42 75.69,28.19 76.33,28.83 R11.1
LED1_PIN
  Bottom 0.254: JP1.5 88.23,25 87.3,25.93 81.08,25.93 80.77,26.24 R15.2
LED2  (via drill 0.35)
  Top 0.254: IC1.55 66.84,15.07 75.06,23.29 v75.06,26.92
  Bottom 0.254: v75.06,26.92 75.06,27.81 74.04,28.83 R12.1
LED2_PIN
  Bottom 0.254: R16.2 85.15,27.62 86.08,26.7 88.8,26.7 89.24,26.26 92.01,26.26 JP1.6
LED3  (via drill 0.35)
  Top 0.254: IC1.54 66.34,15.26 74.28,23.21 74.28,26.91 v74.3,26.92
  Bottom 0.254: v74.3,26.92 74.3,27.51 71.75,30.05 R13.1
LED3_PIN
  Bottom 0.254: R17.2 92.71,31.45 91.97,30.71 91.97,28.78 JP1.3
LED4  (via drill 0.35)
  Top 0.254: IC1.53 65.84,15.41 73.66,23.24 v73.66,26.42
  Bottom 0.254: v73.66,26.42 69.47,30.61 R14.1
LED4_PIN
  Bottom 0.254: R18.2 95.37,28.77 94.14,27.54 JP1.4
MISO
  Top 0.254: IC1.22 66.34,30.26 61.86,34.74 U3.10
MISO_PI
  Top 0.254: IC2.21 59.94,57 59.94,53.8 arc90 60.26,53.48 60.9,53.48 arc-90 61.22,53.17 61.22,52.9 arc-90 60.9,52.59 58.98,52.59 arc90 58.67,52.27 58.67,52 arc90 58.98,51.69 60.9,51.69 arc-90 61.22,51.37 61.22,51.11 arc-90 60.9,50.79 60.26,50.79 arc90 59.94,50.48 59.94,45.67 61.86,43.75 U3.5
MOSI
  Top 0.254: IC1.21 66.84,30.37 62.51,34.7 U3.11
MOSI_PI
  Top 0.254: IC2.19 62.5,56.99 62.5,49.4 arc-90 62.18,49.09 61.42,49.09 arc90 61.1,48.77 61.1,48.42 arc90 61.42,48.1 63.58,48.1 arc-90 63.89,47.79 63.89,47.43 arc-90 63.58,47.12 61.42,47.12 arc90 61.1,46.8 61.1,46.45 arc90 61.42,46.13 62.18,46.13 arc-90 62.5,45.82 62.5,41.75 62.59,41.66 U3.4
N$1
  Bottom 0.406: R05.2 R06.1
N$2
  Bottom 0.406: U2.3 35.14,64.69 R07.1 35.04,65.09 35.58,65.63 35.58,66.63 36.13,67.18 36.96,67.18 37.92,68.15 R03.1 R04.1
N$3
  Bottom 0.406: R08.1 32.11,60.93 | U2.2 40.6,63.42 40.96,63.06 40.96,61.66 40.64,61.34 32.52,61.34 32.11,60.93 | U1.8 30.87,62.16 32.11,60.93
N$5
  Bottom 0.406: R01.1 31.27,69.28 R02.2
N$6  (via drill 0.35)
  Top 0.406: v33.02,62.67 22.28,51.94 22.28,44.69 16.94,39.34 Q01.1
  Bottom 0.406: U2.1 36.98,62.15 36.44,62.69 R07.2 33.03,62.69 v33.02,62.67
N$7
  Bottom 0.406: R03.2 33.2,69.29 R02.1
N$8
  Bottom 0.254: R/W.2 92.08,63.41 90.12,61.45 83.33,61.45 81.59,59.71 81.59,58.3 IC2.3
N$9
  Bottom 0.254: R11.2 76.33,34.02 76.68,34.37 Q11.1
N$10
  Bottom 0.254: R12.2 74.04,35.74 74.37,36.07 81.28,36.07 81.85,35.49 Q12.1
N$11
  Top 0.254: C51.1 81.56,26.2 IC1.98
N$12
  Bottom 0.406: R04.2 45.2,69.3 R05.1
N$13
  Bottom 0.254: R13.2 71.75,35.33 73.38,36.96 83.67,36.96 85.06,35.56 85.06,30.73 85.52,30.28 86.27,30.28 Q13.1
N$14
  Bottom 0.254: R14.2 69.47,35.18 72.17,37.88 84.77,37.88 86.3,36.36 Q14.1
N$18
  Bottom 0.254: Q11.3 80.17,32.17 80.77,31.57 R15.1
N$19
  Bottom 0.254: Q12.3 82.8,31.01 83.06,30.76 R16.1
N$26
  Bottom 0.254: R17.1 91.56,34.23 89.46,32.13 89.46,28.98 88.59,28.11 Q13.3
N$29
  Bottom 0.254: R18.1 95.37,36.59 94.61,37.34 90.5,37.34 89.66,36.5 89.66,33.38 88.46,32.17 Q14.3
N$30  (via drill 0.35)
  Top 0.254: IC1.88 78.84,21.19 80.84,21.19 v81.13,21.48
  Bottom 0.254: v81.13,21.48 81.46,21.14 82.61,21.14 83.08,21.62 R51.1 R52.2
OUTA
  Top 1.27: A2.7 17.97,4.5 A2.8
  Top 2.54: JP2.4 15.15,3.49 16.1,4.45 17.92,4.45 17.97,4.5
OUTB
  Top 1.27: A2.5 17.97,9.78 A2.6
  Top 2.54: JP2.3 12.98,6.99 15.52,9.53 17.72,9.53 17.97,9.78
PWM  (via drill 0.35)
  Top 0.254: IC1.16 69.33,28.3 68.01,26.98 v65.2,26.98
  Bottom 0.254: A2.11 51.46,8.23 50.44,9.25 50.44,15.95 51.61,17.12 60.3,17.12 61.14,17.96 61.14,25.5 62.61,26.98 v65.2,26.98
SCK
  Top 0.254: IC1.20 67.34,30.45 63.16,34.63 U3.12
SCK_PI
  Top 0.254: U3.3 63.16,40.3 62.89,40.03 59.69,40.03 57.4,42.32 57.4,57 IC2.23
SCL  (via drill 0.35)
  Top 0.254: IC1.43 59.21,18.7 v58.42,17.91 | v58.42,17.91
  Bottom 0.254: A1.5 5.7,69.67 24.26,51.12 24.26,34.61 28.93,29.94 54.13,29.94 57,27.08 57,19.33 v58.42,17.91
SDA  (via drill 0.35)
  Top 0.254: IC1.44 59.98,18.2 v59.69,17.91
  Bottom 0.254: A1.4 4.65,72.21 25.3,51.56 25.3,35.44 29.72,31.02 54.58,31.02 57.89,27.71 57.89,19.74 59.03,18.59 59.03,18.57 v59.69,17.91
SENSOR1  (via drill 0.35)
  Top 0.254: IC1.85 81.47,19.7 v81.92,19.25
  Bottom 0.254: JP1.9 84.77,19.92 83.99,19.14 82.02,19.14 v81.92,19.25
SENSOR2  (via drill 0.35)
  Top 0.254: IC1.86 82.5,20.2 v82.68,20.02
  Bottom 0.254: JP1.10 92.06,21.13 90.17,21.13 89.53,20.5 84.58,20.5 84.03,19.95 82.74,19.95 v82.68,20.02
SENSOR3  (via drill 0.35)
  Top 0.254: IC1.87 78.88,20.65 83.31,20.65 v83.34,20.68
  Bottom 0.254: v83.34,20.68 83.97,20.68 84.51,21.21 88.44,21.21 89.69,22.46 JP1.7
SERVO_PWM  (via drill 0.35)
  Top 0.254: IC1.7 73.84,28.38 71.59,26.14 69.22,26.14 v69.19,26.11 | SERVO.3 33.23,19.78 38.46,14.55 60.15,14.55 v61.24,15.65
  Bottom 0.254: v61.24,15.65 62.31,16.71 62.31,24.79 63.64,26.12 69.18,26.12 v69.19,26.11
SS
  Top 0.254: IC1.19 67.84,30.69 63.81,34.72 U3.13
SS_PI
  Top 0.254: U3.2 63.81,40.03 63.09,39.32 59.23,39.32 56.15,42.41 IC2.24
TCK
  Top 0.254: IC1.93 84.74,23.7 87.34,21.09 87.34,12.84 87.05,12.54 | RN1.5 87.05,12.54 | 87.05,12.54 92.19,12.54 JTAG.1
TDI  (via drill 0.35)
  Top 0.254: IC1.90 83.6,22.2 84.22,21.57 84.22,18.7 v84.42,18.5 | RN1.2 89.75,4.92 92.23,2.44 JTAG.9
  Bottom 0.254: v84.42,18.5 83.33,17.42 83.33,5.32 83.73,4.92 RN1.2
TDO  (via drill 0.35)
  Top 0.254: IC1.91 84.1,22.7 84.94,21.85 84.94,19.22 v85.42,18.73 | RN1.4 92.19,10 JTAG.3
  Bottom 0.254: v85.42,18.73 86.05,18.11 87.8,18.11 88.32,17.59 88.32,10.92 87.39,10 RN1.4
TMS  (via drill 0.35)
  Top 0.254: IC1.92 84.37,23.2 85.57,22 85.57,19.8 v86.49,18.88 | RN1.3 92.19,7.46 JTAG.5
  Bottom 0.254: v86.49,18.88 87.9,18.88 88.93,17.84 88.93,8.67 87.72,7.46 RN1.3
VCC_BAT  (via drill 0.35)
  Top 0.406: C61.1 29.23,40.91 29.23,38.02 v29.21,38
  Top 0.61: P1.3 31.91,40.96 C61.1 27.98,40.96 27.13,40.11 | 27.13,27.91 27.13,40.11 | 27.13,40.11 27.13,52.18 v26.1,53.21
  Top 1.27: A2.2 18,18.41 18,19.66 | A2.1 17.97,19.68 18,19.66 | 18,19.66 22.83,19.66 26.17,23 26.17,26.95 27.13,27.91 34.89,27.91 35.77,27.03 SERVO.2
  Top 2.54: 15.45,19.66 18,19.66 | JP2.1 11.2,15.41 15.45,19.66 | C81.+ 9.22,25.89 15.45,19.66
  Bottom 0.406: R51.2 78.42,24.65 77.67,25.4 71.98,25.4 69.62,27.76 62.41,27.76 57.91,32.26 31.55,32.26 29.21,34.59 v29.21,38
  Bottom 0.61: D01.1 25.77,53.54 v26.1,53.21
VCC_BAT_LP  (via drill 0.35)
  Top 0.406: v25.59,67.25 24.83,66.48 v24.83,60.01 24.83,58.69 23.08,56.93 C01.+
  Bottom 0.406: v24.83,60.01 24.82,59.99 D01.3 32.05,58.06 R08.2 33.43,58.01 33.78,58.36 33.78,60.2 34.23,60.64 43.12,60.64 43.86,61.39 U2.8 46.84,62.15 47.34,62.65 C02.1 | R01.2 26.55,68.2 v25.59,67.25
XTAL1  (via drill 0.35)
  Top 0.305: IC1.34 v64.99,23.2 v65,23.19
  Bottom 0.305: v65,23.19 67,23.19 QG1.3

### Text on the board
tNames: Write enable / jumper | CPM_Fahrzeug - Version 2.4 - Oktober 2019 | Raspberry-Pi Zero | Odometer | Servo | BAT+ | BAT- | M+ | M- | Servo / PWM | Servo / Vcc | Servo / GND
